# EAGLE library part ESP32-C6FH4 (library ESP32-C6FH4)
Multiprotocol Modules SMD IC ESP32-C6FH4, RISC-V single-core MCU, 2.4G Wi-Fi 6 & BLE 5.0 combo, 4 MB flash, QFN 32-pin, Source: Datasheet
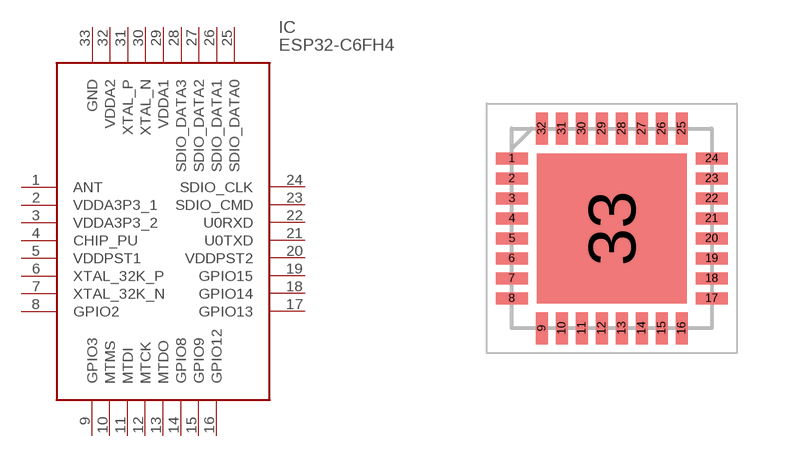
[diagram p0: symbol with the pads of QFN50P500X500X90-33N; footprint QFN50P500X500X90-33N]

Designator prefix IC

## ESP32-C6FH4 (Description: Multiprotocol Modules SMD IC ESP32-C6FH4, RISC-V single-core MCU, 2.4G Wi-Fi 6 & BLE 5.0 combo, 4 MB flash, QFN 32-pin,; Height: 0.9mm; Manufacturer_Name: Espressif Systems; Manufacturer_Part_Number: ESP32-C6FH4; Mouser_Part_Number: 356-ESP32-C6FH4; Mouser_Price-Stock: https://www.mouser.co.uk/ProductDetail/Espressif-Systems/ESP32-C6FH4?qs=Imq1NPwxi77uZvg%252BuAIiXA%3D%3D)  [QFN50P500X500X90-33N]
1  ANT
2  VDDA3P3_1
3  VDDA3P3_2
4  CHIP_PU
5  VDDPST1
6  XTAL_32K_P
7  XTAL_32K_N
8  GPIO2
9  GPIO3
10  MTMS
11  MTDI
12  MTCK
13  MTDO
14  GPIO8
15  GPIO9
16  GPIO12
17  GPIO13
18  GPIO14
19  GPIO15
20  VDDPST2
21  U0TXD
22  U0RXD
23  SDIO_CMD
24  SDIO_CLK
25  SDIO_DATA0
26  SDIO_DATA1
27  SDIO_DATA2
28  SDIO_DATA3
29  VDDA1
30  XTAL_N
31  XTAL_P
32  VDDA2
33  GND

## Footprint QFN50P500X500X90-33N (pad centres in mm)
QFN32A
smd 0.8 x 0.3: 1 -2.5,1.75; 2 -2.5,1.25; 3 -2.5,0.75; 4 -2.5,0.25; 5 -2.5,-0.25; 6 -2.5,-0.75; 7 -2.5,-1.25; 8 -2.5,-1.75; 17 2.5,-1.75; 18 2.5,-1.25; 19 2.5,-0.75; 20 2.5,-0.25; 21 2.5,0.25; 22 2.5,0.75; 23 2.5,1.25; 24 2.5,1.75
smd 0.3 x 0.8: 9 -1.75,-2.5; 10 -1.25,-2.5; 11 -0.75,-2.5; 12 -0.25,-2.5; 13 0.25,-2.5; 14 0.75,-2.5; 15 1.25,-2.5; 16 1.75,-2.5; 25 1.75,2.5; 26 1.25,2.5; 27 0.75,2.5; 28 0.25,2.5; 29 -0.25,2.5; 30 -0.75,2.5; 31 -1.25,2.5; 32 -1.75,2.5
smd 3.75 x 3.75: 33 0,0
